// TwinCAT 3 PLC project TcComPLCProvider
// ProgramVersion: 3.1.4024.0
// libraries:
//   Tc2_Standard, * (Beckhoff Automation GmbH)
//   Tc2_System, * (Beckhoff Automation GmbH)
//   Tc3_Module, * (Beckhoff Automation GmbH)
// project tree:
//   / PlcTask.TcTTO
//   POUs/ FB_Calculation.TcPOU, MAIN.TcPOU
// (motion and I/O tree: see PLC project dyntccomproxy)
// real-time tasks:
//   TASK PlcTask: cycle T#10ms, priority 20, ADS port 350
//   TASK PlcTask1: cycle T#10ms, priority 21, ADS port 351
//   TASK PlcTask2: cycle T#10ms, priority 22, ADS port 352
//   TASK PlcTask3: cycle T#10ms, priority 23, ADS port 353
// variable links:
//   TcComPLCCaller/TcComPLCCaller Instance <-> TcComPLCProvider/TcComPLCProvider Instance
//     PlcTask Inputs/MAIN.fbProxyPLCCalculationTcComModule._objectId <-> PlcTask Outputs/MAIN.fbCalc.objID

CONFIGURATION TcComPLCProvider
    RESOURCE PLC ON TwinCAT3
        TASK PlcTask(INTERVAL := T#10ms, PRIORITY := 22);
        PROGRAM MAIN WITH PlcTask : MAIN;
    END_RESOURCE
END_CONFIGURATION

// ---- POUs/MAIN.TcPOU
PROGRAM MAIN
VAR
	m : UDINT;
	
	fbCalc : FB_Calculation('MAIN.fbCalc');
END_VAR

m := m + 1;

END_PROGRAM

// ---- POUs/FB_Calculation.TcPOU
{attribute 'c++_compatible'}
FUNCTION_BLOCK FB_Calculation EXTENDS TcBaseModuleRegistered IMPLEMENTS I_Calculation

VAR
END_VAR

{attribute 'c++_compatible'}
{attribute 'pack_mode' := '4'}
{attribute 'show'}
{attribute 'minimal_input_size' := '4'}
METHOD Addition : HRESULT
VAR_INPUT
	nIn1	: INT;
	nIn2	: INT;
	nRes	: REFERENCE TO INT;
END_VAR
nRes := nIn1 + nIn2;
END_METHOD

{attribute 'c++_compatible'}
{attribute 'pack_mode' := '4'}
{attribute 'show'}
{attribute 'minimal_input_size' := '4'}
METHOD Subtraction : HRESULT
VAR_INPUT
	nIn1	: INT;
	nIn2	: INT;
	nRes	: REFERENCE TO INT;
END_VAR
nRes := nIn1 - nIn2;
END_METHOD

{attribute 'c++_compatible'}
{attribute 'pack_mode' := '4'}
{attribute 'show'}
{attribute 'minimal_input_size' := '4'}
METHOD TcQueryInterface : HRESULT
VAR_INPUT
	iid	: REFERENCE TO IID;
	pipItf	: POINTER TO PVOID;
END_VAR

VAR
	ipCalc : I_Calculation;
END_VAR
IF GuidsEqual(ADR(iid), ADR(TC_GLOBAL_IID_LIST.IID_I_Calculation)) THEN
	ipCalc := THIS^; 
	pipItf^ := ITCUNKNOWN_TO_PVOID(ipCalc);
	TcAddRef();
	TcQueryInterface := S_OK;
ELSE
	TcQueryInterface := SUPER^.TcQueryInterface(iid, pipItf);
END_IF
END_METHOD

END_FUNCTION_BLOCK
